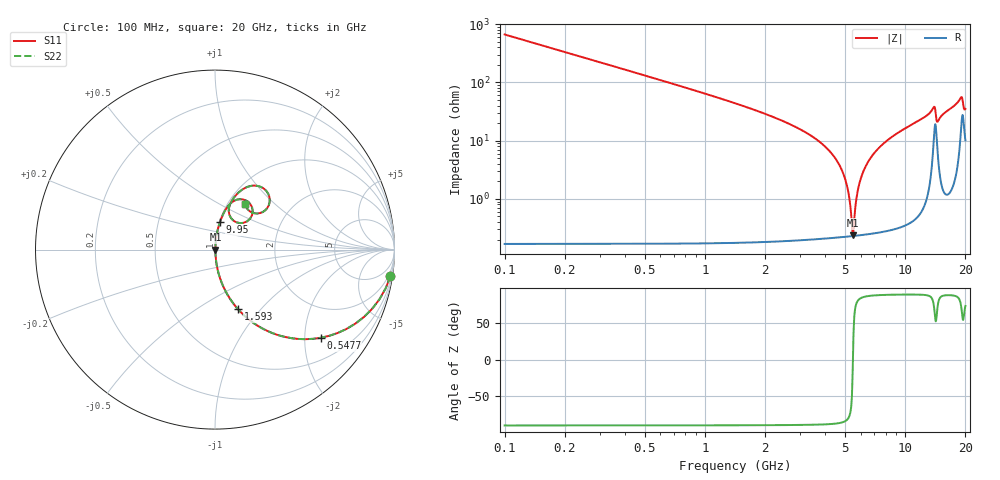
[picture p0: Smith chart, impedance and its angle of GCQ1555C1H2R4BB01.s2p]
!Murata Part Number: GCQ1555C1H2R4BB01
!These Parameters are Measured in Series Mode Connection
!Data Generated on Jan 08, 2026
!  o--ll--o
!Port1  Port2
!  o------o
!Operation Temp=25[degC], DC Bias Voltage=0[V]
!Freq. Start=100[MHz] Stop=20[GHz] 401[Steps]
# Hz S RI R 50
!Freq.(Hz) S11(Real) S11(Imag) S21(Real) S21(Imag) S12(Real) S12(Imag) S22(Real) S22(Imag)
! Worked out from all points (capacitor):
!   401 points, 100 MHz to 20 GHz, reference 50 ohm
!   read as one part in series: C = 2.4 pF near 199.5 MHz
!   lowest |Z| = 238 mohm at 5.473 GHz (marker M1)
!   series resonance near 5.487 GHz, so ESL is about 350 pH
!   S11 on the Smith chart (normalised r, x): 100 MHz: 1, -13; 547.8 MHz: 1.00, -2.40; 1.593 GHz: 1.00, -0.76; 9.95 GHz: 1.01, +0.32; 20 GHz: 1.20, +0.67
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1e8  0.9777 -0.1475  0.0223 0.1475  0.0223 0.1475  0.9777 -0.1475
2.99e8  0.83 -0.3752  0.17 0.3752  0.17 0.3752  0.83 -0.3752
5.4775e8  0.5895 -0.4912  0.4105 0.4912  0.4105 0.4912  0.5895 -0.4912
9.955e8  0.2939 -0.4542  0.7061 0.4542  0.7061 0.4542  0.2939 -0.4542
1.5925e9  0.1283 -0.3321  0.8717 0.3321  0.8717 0.3321  0.1283 -0.3321
3.43325e9  0.0156 -0.1159  0.9844 0.1159  0.9844 0.1159  0.0156 -0.1159
4.876e9  0.00303 -0.0287  0.997 0.0287  0.997 0.0287  0.00303 -0.0287
5.1745e9  0.00245 -0.0142  0.9975 0.0142  0.9975 0.0142  0.00245 -0.0142
5.473e9  0.00229 -0.000629  0.9977 0.000629  0.9977 0.000629  0.00229 -0.000629
5.7715e9  0.00249 0.0123  0.9975 -0.0123  0.9975 -0.0123  0.00249 0.0123
5.9705e9  0.0028 0.0206  0.9972 -0.0206  0.9972 -0.0206  0.0028 0.0206
6.7665e9  0.00517 0.0515  0.9948 -0.0515  0.9948 -0.0515  0.00517 0.0515
8.01025e9  0.0118 0.0947  0.9882 -0.0947  0.9882 -0.0947  0.0118 0.0947
9.9505e9  0.0282 0.1552  0.9718 -0.1552  0.9718 -0.1552  0.0282 0.1552
1.005e10  0.0293 0.1581  0.9708 -0.1581  0.9708 -0.1581  0.0293 0.1581
1.338325e10  0.1026 0.2696  0.8974 -0.2696  0.8974 -0.2696  0.1026 0.2696
1.398025e10  0.1978 0.2522  0.8022 -0.2522  0.8022 -0.2522  0.1978 0.2522
1.447775e10  0.1003 0.1639  0.8997 -0.1639  0.8997 -0.1639  0.1003 0.1639
1.67165e10  0.1167 0.3033  0.8833 -0.3033  0.8833 -0.3033  0.1167 0.3033
1.895525e10  0.2735 0.3386  0.7265 -0.3386  0.7265 -0.3386  0.2735 0.3386
1.95025e10  0.251 0.2035  0.749 -0.2035  0.749 -0.2035  0.251 0.2035
2e10  0.169 0.2531  0.831 -0.2531  0.831 -0.2531  0.169 0.2531
